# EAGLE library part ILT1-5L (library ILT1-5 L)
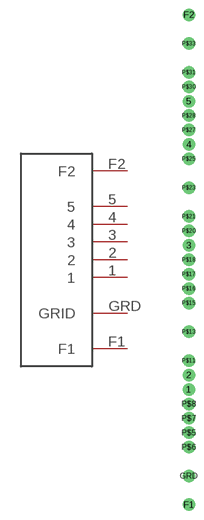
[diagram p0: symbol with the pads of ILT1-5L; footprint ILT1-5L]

Designator prefix -

## ILT1-5L  [ILT1-5L]
1  1
2  2
3  3
4  4
5  5
F1  F1
F2  F2
GRD  GRID

## Footprint ILT1-5L (pad centres in mm)
drill 1.2 pad 2.2: 1 0,20.32; 2 0,22.86; 3 0,45.72; 4 0,63.5; 5 0,71.12; F1 0,0; F2 0,86.36; GRD 0,5.08; P$5 0,12.7; P$6 0,10.16; P$7 0,15.24; P$8 0,17.78; P$11 0,25.4; P$13 0,30.48; P$15 0,35.56; P$16 0,38.1; P$17 0,40.64; P$18 0,43.18; P$20 0,48.26; P$21 0,50.8; P$23 0,55.88; P$25 0,60.96; P$27 0,66.04; P$28 0,68.58; P$30 0,73.66; P$31 0,76.2; P$33 0,81.28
